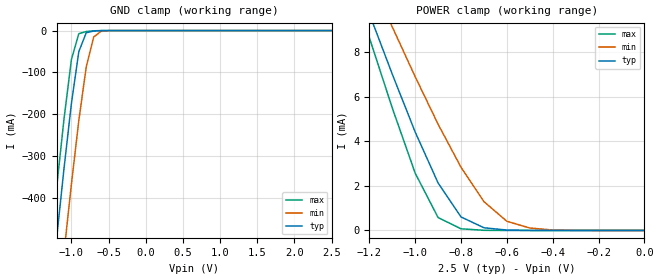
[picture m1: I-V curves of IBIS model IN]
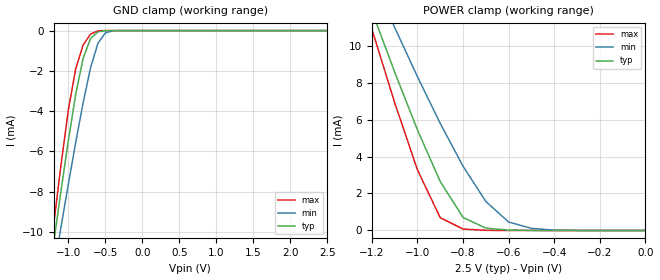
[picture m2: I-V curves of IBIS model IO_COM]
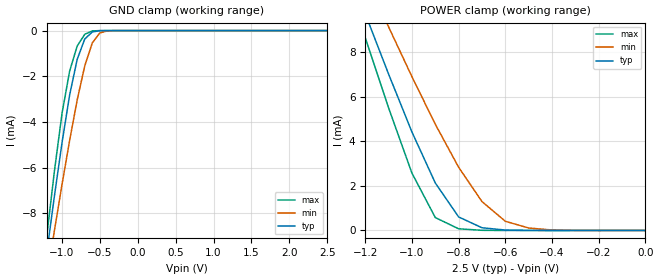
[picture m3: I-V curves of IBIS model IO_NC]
| (C) Copyright DIODES INCORPORATED
| DIODES CORPORATION
| IBIS Model of PI5A23157
| UQFN-10 (ZUA) Package
[IBIS Ver] 3.2
[Comment char] |_char
[File Name] pi5a23157_zua_25v.ibs
[File Rev] 1.0
[Source] File originated at Diodes Incorporated.
[Date] 28/11/24
[Disclaimer]
   All rights reserved
  DIODES Corporation hereby grants the user of
  this IBIS model a non-exclusive, nontransferable license to
  use this IBIS model under the following terms.
  This IBIS model is provided on an "AS IS" basis and Diodes
  makes absolutely no warranty with respect to the information
  contained herein. DIODES DISCLAIMS AND CUSTOMER WAIVES ALL
  WARRANTIES, EXPRESSED OR IMPLIED, INCLUDING WARRANTIES OF
  MERCHANTABILITY OR FITNESS FOR A PARTICULAR PURPOSE. The
  entire risk as to quality and performance is with the customer.
  Accordingly, in no event shall the company be liable for any
  damages, whether in contract or tort, including any lost
  profits or other incidental, consequential, exemplary, or
  punitive damages arising out of the use or application of the
  IBIS model provided in this package. Further, Diodes reserves
  the right to make changes without notice to any product herein
  to improve reliability, function, or design. Diodes does not
  convey any license under patent rights or any other intellectual
  property rights, including those of third parties.
  The user is granted this license only to use the IBIS model
  and is not granted rights to sell, load, rent, lease or license
  the IBIS model in whole or in part, or in modified form to anyone
  other than user. User may modify the IBIS model to suit its specific
  application but rights to derivative works and such modifications
  shall belong to Diodes.
  Diodes is not obligated to provide maintenance or support
  for the licensed IBIS model.
  Contact Diodes at ATTN: APPLICATION ENGINEERING / IBIS MODELS
  1545 Barber Lane Milpitas, CA 95035 USA.
[Component] PI5A23157
[Manufacturer] DIODES CORPORATION
[Package]
|   typ   min   max
R_pkg   50m   45m   55m
L_pkg   1.2n   1.08n   1.32n
C_pkg   0.35p   0.315p   0.385p
[Pin]   signal_name   model_name
1   IN1   IN
2   NO1   IO_NO
3   GND   GND
4   NO2   IO_NO
5   IN2   IN
6   COM2   IO_COM
7   NC2   IO_NC
8   VDD   POWER
9   NC1   IO_NC
10   COM1   IO_COM
[Series Switch Groups]
On   1 /   |NC1 to COM1
On   2 /   |NC2 to COM2
On   3 /   |NO1 to COM1
On   4 /   |NO2 to COM2
On   1 2 /
On   3 4 /
On   1 4 /
On   2 3 /
[Series Pin Mapping]   pin_2   model_name   function_table_group
9   10   SW_25   1
7   6   SW_25   2
2   10   SW_25   3
4   6   SW_25   4
[Model] SW_25
Model_type   Series_switch
Polarity   Non-Inverting
Enable  Active-High
C_comp   8.030pF   7.939pF   8.268pF
[Voltage Range]   2.5   2.3   2.7
[Temperature Range]   25   -40   125
[On]
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[off]
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| Models and submodels in the file (5): IN (Input), IO_COM (Terminator), IO_NC (Terminator), IO_NO (Terminator), SW_25 (Series_switch)
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[Model]   IN
Polarity   Non-Inverting
Model_type   Input
Vinl=0.75
Vinh=1.75
C_comp   1.924pF   1.924pF   1.950pF
[Voltage Range]   2.5   2.3   2.7
[Temperature Range]   25   -40   125
[GND Clamp Reference]   0   0   0
[POWER Clamp Reference]   2.5   2.3   2.7
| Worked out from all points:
|   GND clamp passes 1 mA (typ) near -0.69 V on its own axis
|   POWER clamp passes 1 mA (typ) near -0.83 V on its own axis
[GND_Clamp]
-2.5V     -2.848A    -3.033A    -2.739A
-1.3V     -672mA     -874.9mA   -551.1mA
-1.2V     -498.6mA   -701.3mA   -377.7mA
-1.1V     -330.7mA   -531.4mA   -212.2mA
-1V       -174.4mA   -367.4mA   -69.35mA
-900mV    -50.06mA   -214.6mA   -7.417mA
-800mV    -5.194mA   -86.41mA   -2.283mA
-700mV    -1.045mA   -15.38mA   -516.4uA
-600mV    -172uA     -1.514mA   -42.54uA
2.5V      91.3pA     970.8pA    90pA
[Power_Clamp]
|   X   TYP   MIN   MAX
-2.5V     36.63mA    30.99mA    40.56mA
-1.3V     12.45mA    13.71mA    11.79mA
-1.2V     9.728mA    11.42mA    8.659mA
-1.1V     7.02mA     9.139mA    5.502mA
-1V       4.42mA     6.903mA    2.574mA
-900mV    2.132mA    4.769mA    579.9uA
-800mV    606.9uA    2.838mA    75.2uA
-700mV    121.6uA    1.296mA    7.847uA
-600mV    18.95uA    412.9uA    573.1nA
-500mV    1.921uA    111uA      23.52nA
-400mV    132.9nA    20.24uA    1.549nA
0V        377.6pA    3.593nA    399.6pA
[Model]   IO_COM
Model_type   Terminator
C_comp   8.030pF   7.939pF   8.268pF
[Voltage Range]   2.5   2.3   2.7
[Temperature Range]   25   -40   125
[GND Clamp Reference]   0   0   0
[POWER Clamp Reference]   2.5   2.3   2.7
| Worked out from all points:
|   GND clamp passes 1 mA (typ) near -0.76 V on its own axis
|   POWER clamp passes 1 mA (typ) near -0.82 V on its own axis
[GND_Clamp]
-2.5V     -3.187A    -3.87A     -2.731A
-1.3V     -13.25mA   -14.77mA   -12.81mA
-1.2V     -10.6mA    -12.01mA   -9.718mA
-1.1V     -7.997mA   -9.789mA   -6.708mA
-1V       -5.476mA   -7.643mA   -3.954mA
-900mV    -3.167mA   -5.561mA   -1.899mA
-800mV    -1.385mA   -3.592mA   -718.3uA
-700mV    -401.3uA   -1.861mA   -175uA
-600mV    -64.78uA   -636uA     -15.81uA
-500mV    -5.832uA   -117.2uA   -626.1nA
-400mV    -349.1nA   -12.1uA    -14.84nA
2.5V      503.6pA    231.8nA    278.5pA
[Power_Clamp]
-2.5V     65.73mA    56.47mA    73.27mA
-1.2V     11.87mA    13.75mA    10.89mA
-1.1V     8.566mA    10.98mA    6.91mA
-1V       5.435mA    8.315mA    3.275mA
-900mV    2.645mA    5.787mA    688.9uA
-800mV    704.7uA    3.472mA    77.16uA
-700mV    125.6uA    1.567mA    7.958uA
-600mV    19.27uA    457.1uA    579.8nA
-500mV    1.945uA    114.8uA    23.83nA
-400mV    134.6nA    20.64uA    1.571nA
0V        502.2pA    3.828nA    527pA
[Model]   IO_NC
Model_type   Terminator
C_comp   2.989pF   2.956pF   3.111pF
[Voltage Range]   2.5   2.3   2.7
[Temperature Range]   25   -40   125
[GND Clamp Reference]   0   0   0
[POWER Clamp Reference]   2.5   2.3   2.7
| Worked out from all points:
|   GND clamp passes 1 mA (typ) near -0.77 V on its own axis
|   POWER clamp passes 1 mA (typ) near -0.83 V on its own axis
[GND_Clamp]
-2.5V     -1.685A    -2.018A    -1.463A
-1.2V     -9.674mA   -10.81mA   -8.944mA
-1.1V     -7.224mA   -8.733mA   -6.127mA
-1V       -4.897mA   -6.727mA   -3.616mA
-900mV    -2.821mA   -4.809mA   -1.777mA
-800mV    -1.257mA   -3.037mA   -673.9uA
-700mV    -367.7uA   -1.543mA   -161.9uA
-600mV    -59.25uA   -533uA     -14.42uA
-500mV    -5.324uA   -102.4uA   -563.2nA
-400mV    -316nA     -10.83uA   -13.24nA
2.5V      376.1pA    228.5nA    251.9pA
[Power_Clamp]
-2.5V     36.63mA    31.09mA    40.56mA
-1.3V     12.45mA    13.71mA    11.79mA
-1.2V     9.728mA    11.42mA    8.659mA
-1.1V     7.02mA     9.139mA    5.502mA
-1V       4.42mA     6.903mA    2.574mA
-900mV    2.132mA    4.769mA    579.9uA
-800mV    606.9uA    2.838mA    75.2uA
-700mV    121.6uA    1.296mA    7.847uA
-600mV    18.95uA    412.9uA    573.1nA
-500mV    1.921uA    111uA      23.52nA
-400mV    132.9nA    20.24uA    1.545nA
0V        377.4pA    3.594nA    399.7pA
